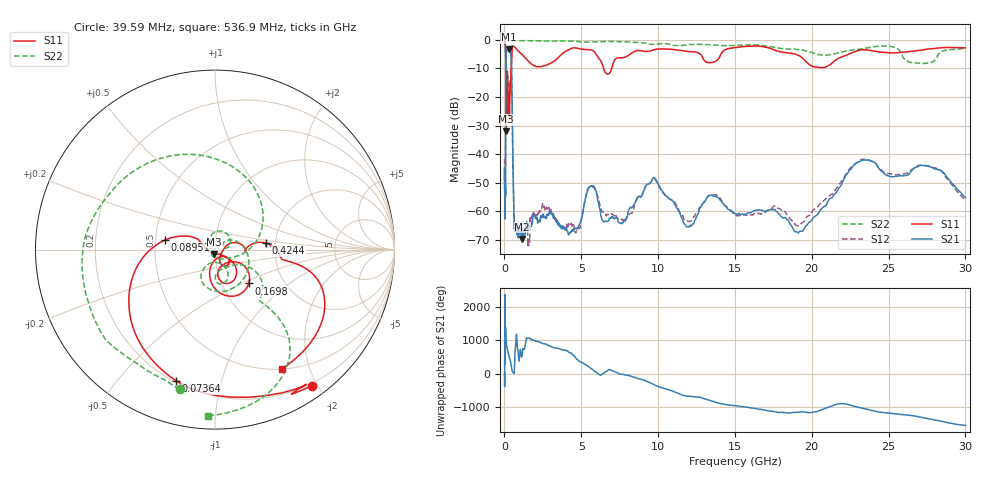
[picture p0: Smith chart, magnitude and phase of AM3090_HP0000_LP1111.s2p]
! Date/Time: Thu, Feb 28, 2019 1:53 PM
! Network Analyzer: Agilent Technologies E8364B Rev: A.07.50.67
! Sweep from 0.010 to 30.000 GHz, 1601 Points, Sweep Type: LOG
! Power Supply: 5.022 V, 0.002 A
# Hz S DB R 50
!freq MagS11 AngS11 MagS21 AngS21 MagS12 AngS12 MagS22 AngS22
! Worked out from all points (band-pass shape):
!   1601 points, 10 MHz to 30 GHz, reference 50 ohm
!   highest |S21| = -3.30 dB at 263.8 MHz (marker M1); lowest = -69.7 dB at 1.16 GHz (marker M2)
!   |S21| within 3 dB of the highest: 101.1 MHz to 441.4 MHz (340.2 MHz wide, 125 % of centre)
!   lowest |S11| = -31.9 dB at 97.94 MHz (marker M3), VSWR 1.05, Z = 49.5 - j2.46 ohm
!   |S11| at or under -10 dB: 88.95 MHz to 429.2 MHz (340.3 MHz wide, 131 % of centre); 6.455 GHz to 6.98 GHz (525.2 MHz wide, 7.82 % of centre)
!   |S22| runs from -31.4 to -0.2 dB; largest |S21 - S12| = 0.013
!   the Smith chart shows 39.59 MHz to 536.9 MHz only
!   S11 on the Smith chart (normalised r, x): 39.59 MHz: 0.17, -1.93; 73.64 MHz: 0.21, -0.73; 89.51 MHz: 0.56, +0.07; 169.8 MHz: 1.34, -0.54; 424.4 MHz: 1.79, +0.14; 536.9 MHz: 0.50, -1.59
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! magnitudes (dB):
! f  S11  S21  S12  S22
! 10 MHz  -0.3  -45.2  -41.6  -0.7
! 38.04 MHz  -0.5  -60.8  -61.4  -1.8
! 39.59 MHz  -0.6  -58.8  -62.0  -1.9
! 73.64 MHz  -2.4  -45.2  -46.9  -4.2
! 89.51 MHz  -11.0  -15.0  -14.9  -12.2
! 97.94 MHz  -31.9  -7.2  -7.2  -31.2
! 113.2 MHz  -14.1  -4.8  -4.8  -19.4
! 144.7 MHz  -18.5  -3.6  -3.5  -24.4
! 169.8 MHz  -11.5  -3.5  -3.4  -14.5
! 263.8 MHz  -21.5  -3.3  -3.3  -17.2
! 424.4 MHz  -10.8  -5.3  -5.3  -11.2
! 536.9 MHz  -2.4  -38.3  -38.0  -0.7
! 550.5 MHz  -2.3  -43.0  -42.6  -0.5
! 655.8 MHz  -2.5  -65.5  -65.8  -0.2
! 1.16 GHz  -5.2  -69.7  -66.4  -0.3
! 2.084 GHz  -9.4  -62.2  -61.3  -0.3
! 5.668 GHz  -3.6  -51.0  -51.4  -0.8
! 7.926 GHz  -5.9  -62.4  -62.7  -0.7
! 9.634 GHz  -3.6  -48.5  -48.6  -1.6
! 19.31 GHz  -6.0  -66.9  -64.2  -3.5
! 23.36 GHz  -3.5  -42.0  -41.8  -3.1
! 30 GHz  -2.8  -55.1  -56.2  -3.1
